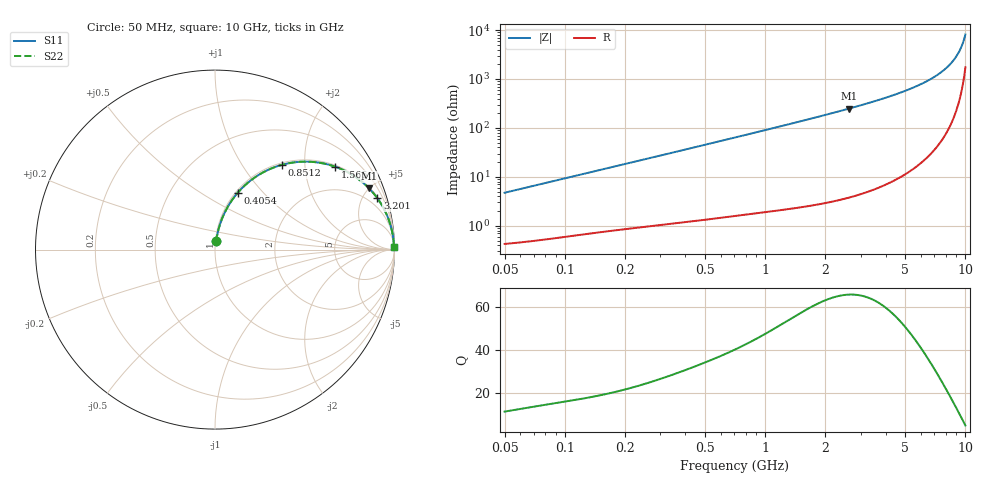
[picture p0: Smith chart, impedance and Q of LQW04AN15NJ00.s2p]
!Murata Part Number: LQW04AN15NJ00
!These Parameters are Measured in Series Mode Connection
!  o--[Z]--o
!Port1  Port2
!  o-------o
!Freq. Start=50[MHz] Stop=10[GHz], 401[Steps]
# Hz S RI R 50
!Freq.(Hz)	S 11(Real)	S 11(Imag)	S 21(Real)	S 21(Imag)	S 12(Real)	S 12(Imag)	S 22(Real)	S 22(Imag)
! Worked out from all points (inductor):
!   401 points, 50 MHz to 10 GHz, reference 50 ohm
!   read as one part in series: L = 15 nH near 51.34 MHz
!   highest Q = 65.9 at 2.624 GHz (marker M1), where L = 15.1 nH
!   S11 on the Smith chart (normalised r, x): 50 MHz: 1.01, +0.09; 405.4 MHz: 1.02, +0.73; 851.2 MHz: 1.03, +1.54; 1.565 GHz: 1.05, +2.86; 3.201 GHz: 1.10, +6.27; 10 GHz: open
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5e7  0.00645 0.0468  0.9935 -0.0468  0.9935 -0.0468  0.00645 0.0468
1.214486e8  0.0189 0.1099  0.9811 -0.1099  0.9811 -0.1099  0.0189 0.1099
1.905373e8  0.0373 0.1671  0.9627 -0.1671  0.9627 -0.1671  0.0373 0.1671
2.949953e8  0.0755 0.2458  0.9245 -0.2458  0.9245 -0.2458  0.0755 0.2458
4.053936e8  0.1269 0.317  0.8731 -0.317  0.8731 -0.317  0.1269 0.317
5.354032e8  0.1966 0.3835  0.8034 -0.3835  0.8034 -0.3835  0.1966 0.3835
7.071068e8  0.2941 0.4434  0.7059 -0.4434  0.7059 -0.4434  0.2941 0.4434
8.511793e8  0.3739 0.4726  0.6261 -0.4726  0.6261 -0.4726  0.3739 0.4726
1.154331e9  0.5213 0.4898  0.4787 -0.4898  0.4787 -0.4898  0.5213 0.4898
1.565451e9  0.6682 0.4624  0.3318 -0.4624  0.3318 -0.4624  0.6682 0.4624
1.717543e9  0.709 0.446  0.291 -0.446  0.291 -0.446  0.709 0.446
2.624158e9  0.8573 0.3423  0.1427 -0.3423  0.1427 -0.3423  0.8573 0.3423
3.200947e9  0.904 0.2869  0.096 -0.2869  0.096 -0.2869  0.904 0.2869
4.171863e9  0.9474 0.2148  0.0526 -0.2148  0.0526 -0.2148  0.9474 0.2148
5.088839e9  0.9688 0.164  0.0312 -0.164  0.0312 -0.164  0.9688 0.164
5.965537e9  0.9808 0.1257  0.0192 -0.1257  0.0192 -0.1257  0.9808 0.1257
6.810442e9  0.9879 0.0953  0.0121 -0.0953  0.0121 -0.0953  0.9879 0.0953
7.672705e9  0.9924 0.0688  0.00758 -0.0688  0.00758 -0.0688  0.9924 0.0688
8.418147e9  0.9949 0.0487  0.00511 -0.0487  0.00511 -0.0487  0.9949 0.0487
8.994549e9  0.9961 0.0345  0.00387 -0.0345  0.00387 -0.0345  0.9961 0.0345
9.359165e9  0.9967 0.026  0.00333 -0.026  0.00333 -0.026  0.9967 0.026
1e10  0.9972 0.0119  0.00276 -0.0119  0.00276 -0.0119  0.9972 0.0119
